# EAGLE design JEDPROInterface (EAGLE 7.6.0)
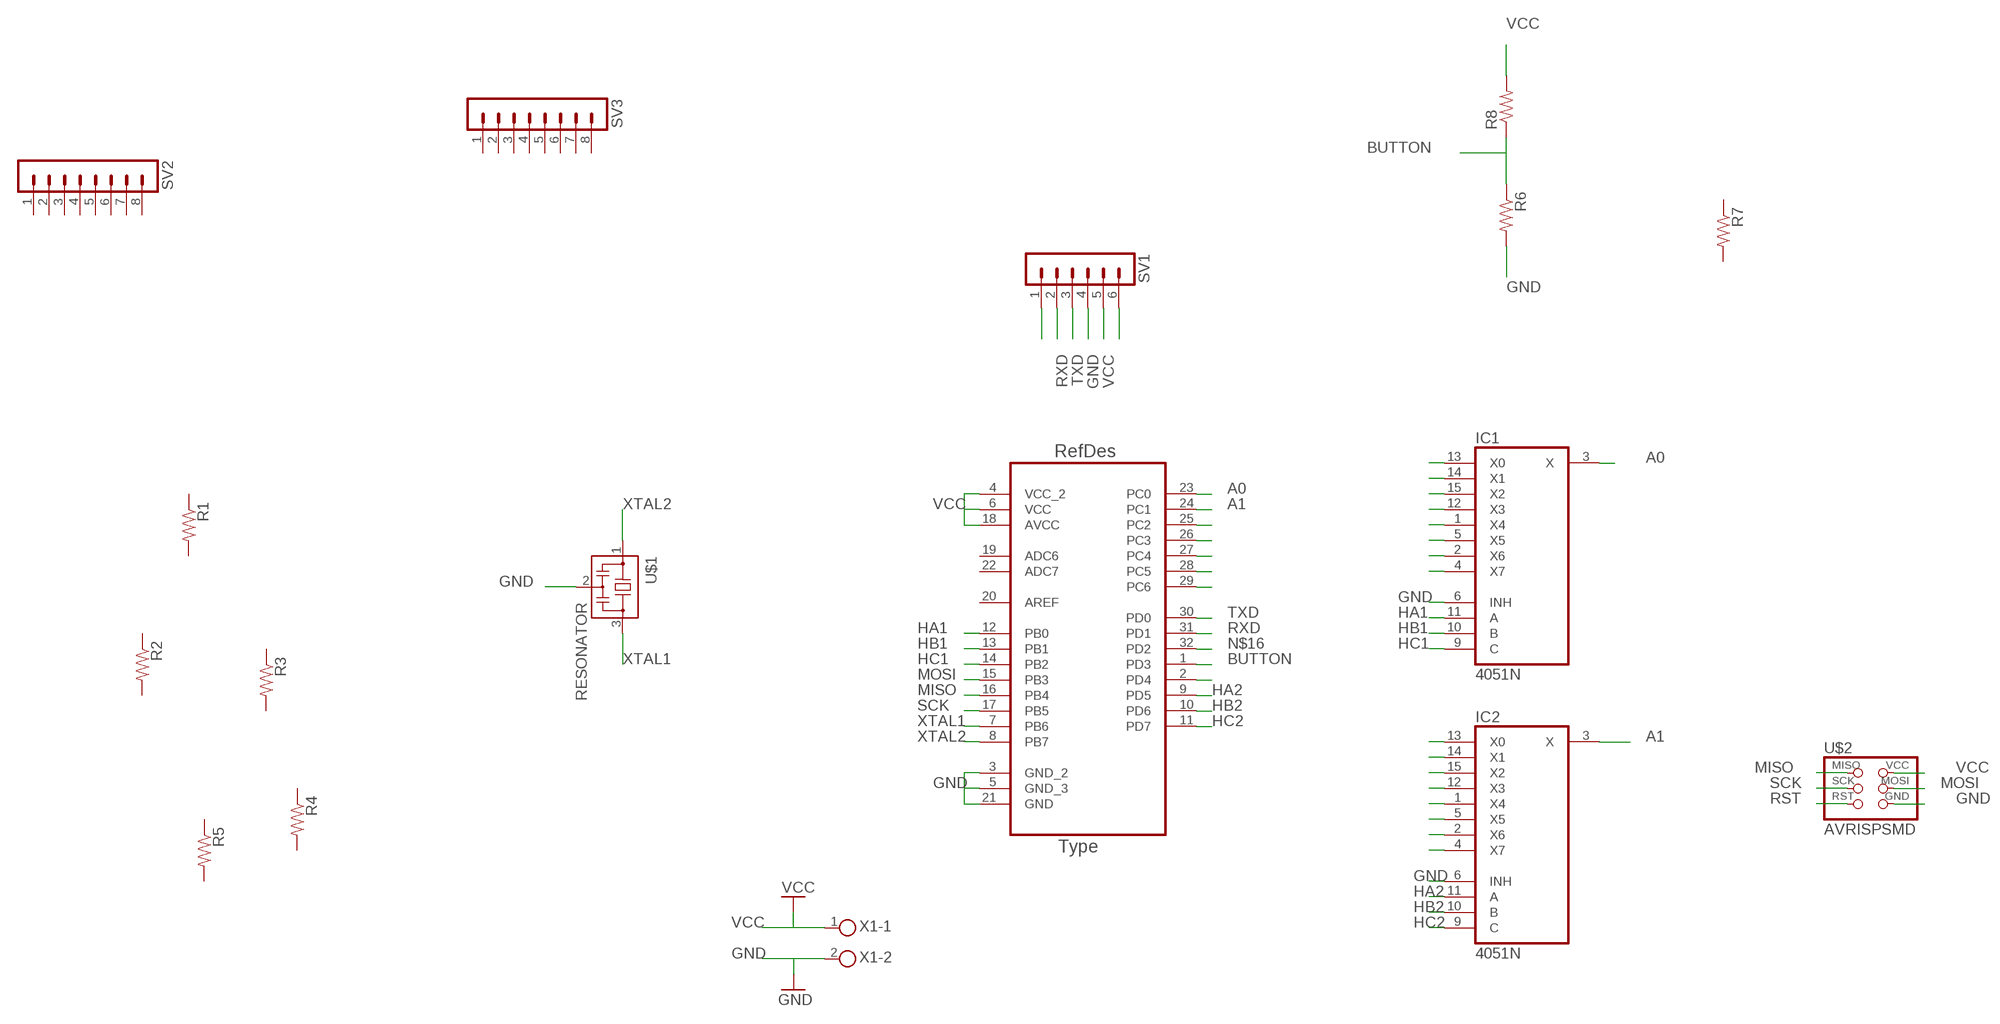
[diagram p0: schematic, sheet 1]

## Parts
IC1  4051N  [DIL16]
IC2  4051N  [DIL16]
R1  RES-US1206FAB  [R1206FAB]
R2  RES-US1206FAB  [R1206FAB]
R3  RES-US1206FAB  [R1206FAB]
R4  RES-US1206FAB  [R1206FAB]
R5  RES-US1206FAB  [R1206FAB]
R6  RES-US1206FAB  [R1206FAB]
R7  RES-US1206FAB  [R1206FAB]
R8  R-US_0204/7  [0204/7]
SV1  MA06-1  [MA06-1]
SV2  MA08-1  [MA08-1]
SV3  MA08-1  [MA08-1]
U1  ATMEGA328P-AU  [QFP80P900X900X120-32N]
U$1  RESONATOR  [EFOBM]
U$2  AVRISPSMD  [2X03SMD]
X1  AKL59-02  [2POL35]

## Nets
A0: IC1.3(X) U1.23(PC0)
A1: IC2.3(X) U1.24(PC1)
BUTTON: R6.1 R8.1 U1.1(PD3)
GND: IC1.6(INH) IC2.6(INH) R6.2 SV1.4 U1.3(GND_2) U1.5(GND_3) U1.21(GND) U$1.2 U$2.6(GND) X1.2
HA1: IC1.11(A) U1.12(PB0)
HA2: IC2.11(A) U1.9(PD5)
HB1: IC1.10(B) U1.13(PB1)
HB2: IC2.10(B) U1.10(PD6)
HC1: IC1.9(C) U1.14(PB2)
HC2: IC2.9(C) U1.11(PD7)
MISO: U1.16(PB4) U$2.1(MISO)
MOSI: U1.15(PB3) U$2.4(MOSI)
N$1: SV1.1
N$2: U1.28(PC5)
N$3: U1.27(PC4)
N$4: U1.26(PC3)
N$5: IC2.4(X7)
N$6: IC2.2(X6)
N$7: IC2.5(X5)
N$8: IC2.1(X4)
N$9: IC2.12(X3)
N$10: IC2.15(X2)
N$11: IC2.14(X1)
N$12: IC2.13(X0)
N$13: U1.25(PC2)
N$16: U1.32(PD2)
N$18: IC1.4(X7)
N$19: IC1.2(X6)
N$20: IC1.5(X5)
N$21: IC1.1(X4)
N$22: IC1.12(X3)
N$23: IC1.15(X2)
N$24: IC1.14(X1)
N$25: IC1.13(X0)
N$26: U1.2(PD4)
N$31: SV1.6
RST: U1.29(PC6) U$2.5(RST)
RXD: SV1.2 U1.31(PD1)
SCK: U1.17(PB5) U$2.3(SCK)
TXD: SV1.3 U1.30(PD0)
VCC: R8.2 SV1.5 U1.4(VCC_2) U1.6(VCC) U1.18(AVCC) U$2.2(VCC) X1.1
XTAL1: U1.7(PB6) U$1.3
XTAL2: U1.8(PB7) U$1.1
Unconnected: R1.1 R1.2 R2.1 R2.2 R3.1 R3.2 R4.1 R4.2 R5.1 R5.2 R7.1 R7.2 SV2.1 SV2.2 SV2.3 SV2.4 SV2.5 SV2.6 SV2.7 SV2.8 SV3.1 SV3.2 SV3.3 SV3.4 SV3.5 SV3.6 SV3.7 SV3.8 U1.19(ADC6) U1.20(AREF) U1.22(ADC7)

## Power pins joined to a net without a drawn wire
GND: IC1.8(GND) IC2.8(GND)
VCC: IC1.16(VCC) IC2.16(VCC)
VEE: IC1.7(VEE) IC2.7(VEE)

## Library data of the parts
IC1 IC2 = 40xx:4051: 8-channel ANALOG MULTIPLEXER
R1-R7 = fab:RES-US: Resistor (US Symbol)
R8 = rcl:R-US_: RESISTOR, American symbol
SV1 = con-lstb:MA06-1: PIN HEADER; OC_FARNELL: unknown; OC_NEWARK: unknown
SV2 SV3 = con-lstb:MA08-1: PIN HEADER; OC_FARNELL: unknown; OC_NEWARK: unknown
U1 = Atmel-ATMEGA328P-AU:ATMEGA328P-AU; DESCRIPTION: 8-bit Microcontroller with In-System Programmable Flash; MPN: ATMEGA328P-AU; OC_FARNELL: 1715486; OC_NEWARK: 14R4631; PACKAGE: TQFP-32; SUPPLIER: Atmel
U$1 = fab:RESONATOR
U$2 = fab:AVRISP
X1 = con-ria-59:AKL59-02: RIA Anschlussklemme Typ 59, Raster 3,5 mm, Polzahl 2

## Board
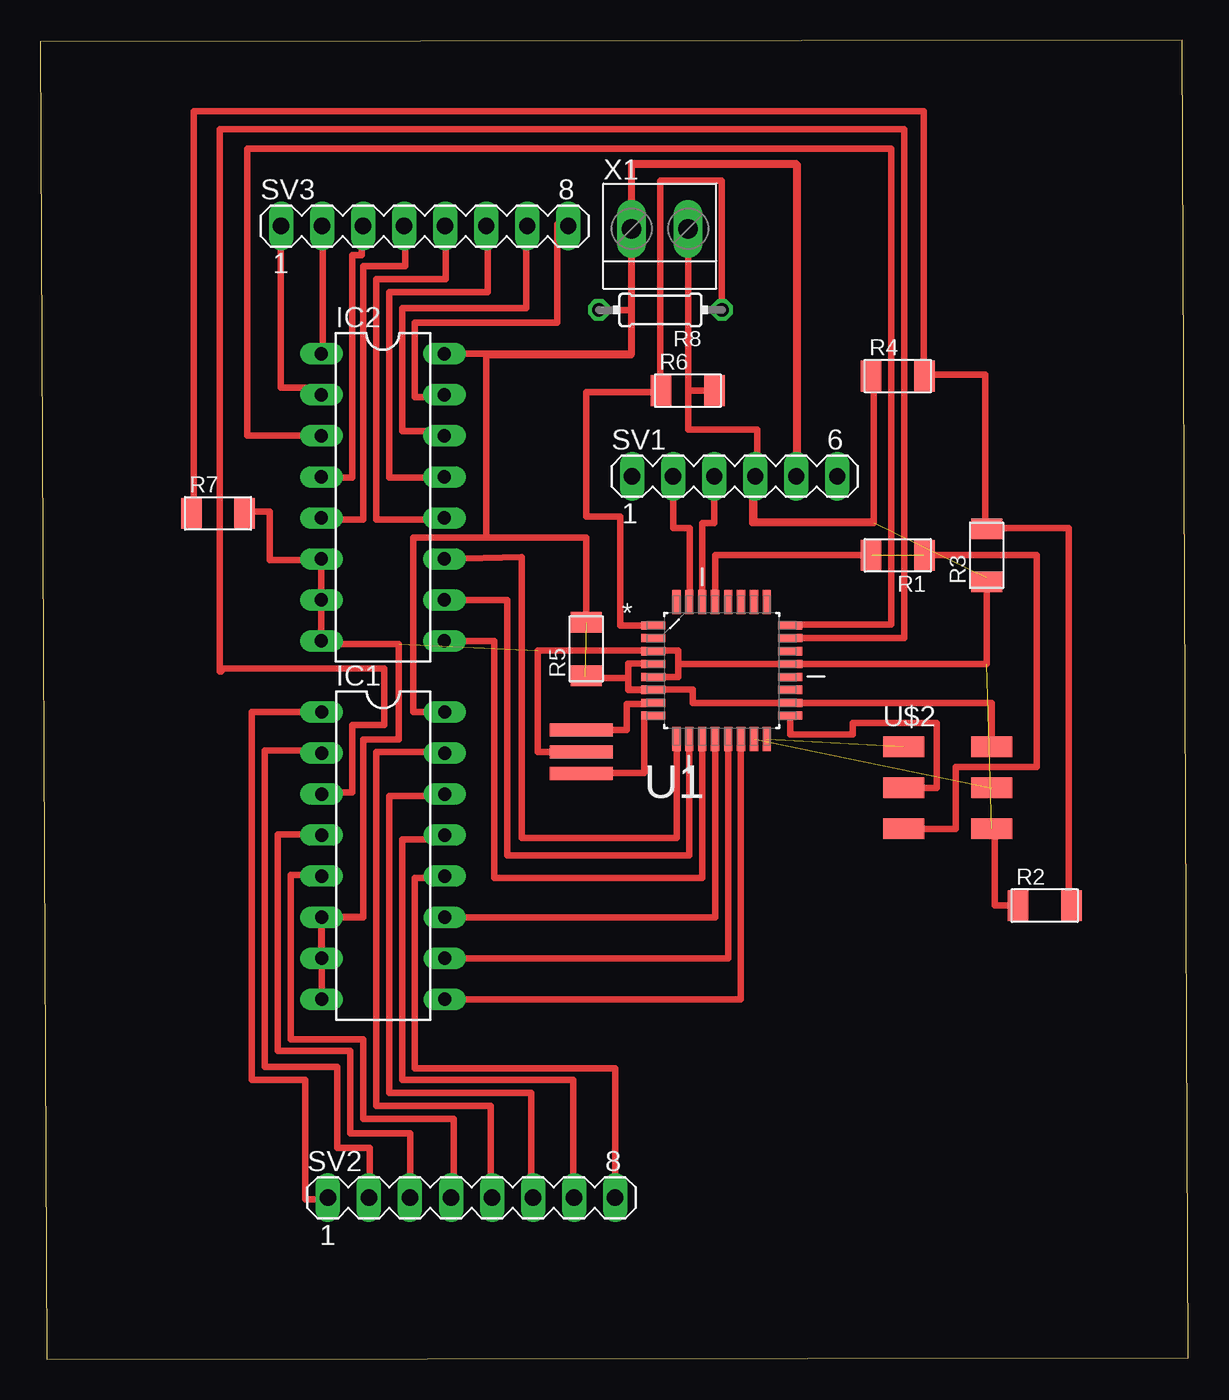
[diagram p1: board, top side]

Size 71.1 x 81.7 mm. Coordinates in mm from the lower left corner, seen from the top.
Outline: 0.4,0 71.1,0.1 70.7,81.7 0,81.6 0.4,0
Copper layers (1*16): Top 0.035mm / dielectric 1.5mm / Bottom 0.035mm
Design rules "default": minimum track width 10mil, minimum drill 24mil, track to track 8mil, track to pad 8mil, pad to pad 8mil, via to via 8mil, smd to smd 8mil, copper to edge 40mil, drill to drill 8mil, minimum pad ring 10mil, minimum via ring 8mil, stop-mask expansion 4mil, vias tented up to drill 0mil, thermal gap 10mil

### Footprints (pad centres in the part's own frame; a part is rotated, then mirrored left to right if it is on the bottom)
DIL16 = drill 0.813 long: 1 -8.89,-3.81; 2 -6.35,-3.81; 3 -3.81,-3.81; 4 -1.27,-3.81; 5 1.27,-3.81; 6 3.81,-3.81; 7 6.35,-3.81; 8 8.89,-3.81; 9 8.89,3.81; 10 6.35,3.81; 11 3.81,3.81; 12 1.27,3.81; 13 -1.27,3.81; 14 -3.81,3.81; 15 -6.35,3.81; 16 -8.89,3.81
R1206FAB = smd 1.27 x 1.905: 1 -1.651,0; 2 1.651,0
0204/7 = drill 0.813 octagon: 1 -3.81,0; 2 3.81,0
MA06-1 = drill 1.016 long: 1 -6.35,0; 2 -3.81,0; 3 -1.27,0; 4 1.27,0; 5 3.81,0; 6 6.35,0
MA08-1 = drill 1.016 long: 1 -8.89,0; 2 -6.35,0; 3 -3.81,0; 4 -1.27,0; 5 1.27,0; 6 3.81,0; 7 6.35,0; 8 8.89,0
QFP80P900X900X120-32N = smd 1.473 x 0.508: 1 -4.242,2.794; 2 -4.242,2.007; 3 -4.242,1.194; 4 -4.242,0.406; 5 -4.242,-0.406; 6 -4.242,-1.194; 7 -4.242,-2.007; 8 -4.242,-2.794; 17 4.242,-2.794; 18 4.242,-2.007; 19 4.242,-1.194; 20 4.242,-0.406; 21 4.242,0.406; 22 4.242,1.194; 23 4.242,2.007; 24 4.242,2.794 | smd 0.508 x 1.473: 9 -2.794,-4.242; 10 -2.007,-4.242; 11 -1.194,-4.242; 12 -0.406,-4.242; 13 0.406,-4.242; 14 1.194,-4.242; 15 2.007,-4.242; 16 2.794,-4.242; 25 2.794,4.242; 26 2.007,4.242; 27 1.194,4.242; 28 0.406,4.242; 29 -0.406,4.242; 30 -1.194,4.242; 31 -2.007,4.242; 32 -2.794,4.242
EFOBM = smd 0.8 x 3.9: 1 -1.35,0; 2 0,0; 3 1.35,0
2X03SMD = smd 2.54 x 1.27: 1 -2.54,2.54; 2 2.92,2.54; 3 -2.54,0; 4 2.92,0; 5 -2.54,-2.54; 6 2.92,-2.54
2POL35 = drill 1.2 long: 1 -1.75,0; 2 1.75,0

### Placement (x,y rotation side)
IC1  21.23,31.19 270 top
IC2  21.21,53.39 270 top
R1  53.1,49.8 180 top
R2  62.2,28.1 0 top
R3  58.6,49.8 90 top
R4  53.1,60.9 0 top
R5  33.8,44 90 top
R6  40.1,60 0 top
R7  11,52.4 0 top
R8  38.4,65 180 top
SV1  43,54.7 0 top
SV2  26.7,10 0 top
SV3  23.8,70.2 0 top
U1  42.19,42.66 0 top
U$1  33.5,37.62 90 top
U$2  56,35.4 0 top
X1  38.36,70.03 0 top

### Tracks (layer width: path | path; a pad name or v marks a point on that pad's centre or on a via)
A0
  Top 0.406: U1.23 53.5,44.67 53.5,76.2 11.1,76.2 11.1,42.6 11.2,42.6 11.2,42.8 21.3,42.8 21.3,39.3 19.3,39.3 19.3,35.1 17.42,35.1 IC1.3
A1
  Top 0.406: IC2.3 12.8,57.2 12.8,75 52.7,75 52.7,45.5 46.43,45.5 U1.24
BUTTON
  Top 0.406: U1.1 35.9,45.45 35.9,52.2 33.8,52.2 33.8,59.9 38.45,59.9 R6.1 38.4,60 38.4,73 42.21,73 R8.1
GND  (3 unrouted)
  Top 0.406: IC1.8 IC1.6 20,27.38 20,38.4 22.2,38.4 22.2,44.3 17.4,44.3 IC2.8 17.4,49.5 | 17.4,49.5 IC2.6 | U1.5 39.5,42.25 39.5,43.07 | 39.5,43.07 39.5,43.9 37.95,43.9 | 39.5,43.07 U1.21 58.6,43.07 58.6,48.4 | U$1.2 30.8,37.62 30.8,43.9 37.95,43.9 | 37.95,43.9 U1.3 | SV1.4 44.4,54.7 44.4,57.6 40.11,57.6 40.11,60 | 40.11,60 X1.2 | SV1.4 44.1,54.7 44.1,51.8 51.6,51.8 51.6,51.9 | 51.6,51.9 51.6,61 | SV1.4 44.2,54.7 44.2,51.9 51.6,51.9 | 17.4,49.5 14.2,49.5 14.2,52.5 12.5,52.5 12.5,52.6 | R6.2 40.11,60
HA1
  Top 0.406: IC1.11 41.78,27.38 U1.12
HA2
  Top 0.406: IC2.11 29.8,49.68 29.8,32.3 39.4,32.3 U1.9
HB1
  Top 0.406: IC1.10 42.6,24.84 U1.13
HB2
  Top 0.406: IC2.10 28.9,47.04 28.9,31.2 40.18,31.2 U1.10
HC1
  Top 0.406: IC1.9 43.38,22.3 U1.14
HC2
  Top 0.406: IC2.9 28.1,44.5 28.1,29.8 41,29.8 U1.11
MISO  (1 unrouted)
MOSI  (1 unrouted)
N$14
  Top 0.406: 17.5,30 15.5,30 15.5,19.8 20,19.8 20,14.9 25.6,14.9 25.6,9.9
N$15
  Top 0.406: 25.2,32.2 22.4,32.2 22.4,17.3 33,17.3 33,10
N$27
  Top 0.406: 24.9,34.9 21.6,34.9 21.6,16.5 30.4,16.5 30.4,13.8 30.4,13.7 30.4,10.1
N$28
  Top 0.406: 25,37.6 20.8,37.6 20.8,15.7 27.9,15.7 27.9,13.5
N$29
  Top 0.406: 59.1,32.5 59.1,28.1 60.6,28.1 60.6,28
N$30
  Top 0.406: 64.2,28.2 63.7,28.2 63.7,51.5 58.6,51.5 58.6,51.7
N$33
  Top 0.406: 25.2,59.6 23.2,59.6 23.2,64.2 32,64.2 32,70.1 32,70.2 32,70.3 32.7,70.3
N$34
  Top 0.406: 25.2,57.5 22.4,57.5 22.4,65.1 30.1,65.1 30.1,70.2
N$35
  Top 0.406: 25.1,54.6 21.6,54.6 21.6,66.1 27.7,66.1 27.7,70.2
N$36
  Top 0.406: 25,52 20.8,52 20.8,66.9 25.1,66.9 25.1,70.2
N$37
  Top 0.406: 17.3,52 20,52 20,67.7 22.6,67.7 22.6,70
N$38
  Top 0.406: 17.4,54.6 19.3,54.6 19.3,68.4 19.9,68.4 19.9,70.2
N$39
  Top 0.406: 17.5,62.3 17.5,70.4
N$40
  Top 0.406: 17.5,60.2 14.9,60.2 14.9,70.5
N$41
  Top 0.406: 25,29.8 23.2,29.8 23.2,18 35.6,18 35.6,13.7 35.6,13.6 35.6,9.9
N$42
  Top 0.406: 27.9,13.4 27.9,9.9
N$43
  Top 0.406: 17.6,32.5 14.7,32.5 14.7,19.1 19.2,19.1 19.2,14 22.9,14 22.9,10
N$44
  Top 0.406: 17.6,37.7 13.9,37.7 13.9,18.1 18.4,18.1 18.4,13.1 20.4,13.1 20.4,10.1
N$45
  Top 0.406: 17.4,40.1 13.1,40.1 13.1,17.3 16.4,17.3 16.4,9.9 17.7,9.9 17.7,10.1
N$46
  Top 0.406: 9.5,53 9.5,77.3 54.7,77.3 54.7,61 58.5,61 58.5,51.4 58.7,51.4
RST  (1 unrouted)
  Top 0.406: U$2.5 56.7,32.86 56.7,36.7 61.7,36.7 61.7,49.8 54.7,49.8 | U1.29 41.78,49.8 51.5,49.8
RXD
  Top 0.406: U1.31 40.2,46.9 40.2,51.5 39.19,51.5 SV1.2
SCK
  Top 0.406: U$2.3 55.5,35.4 55.5,39.4 50.3,39.4 50.3,38.7 46.43,38.7 U1.17
TXD
  Top 0.406: U1.30 41,51.8 41.73,51.8 SV1.3
VCC  (1 unrouted)
  Top 0.406: U$2.2 58.92,40.65 U1.18 40.4,40.65 40.4,41.5 37.95,41.5 | 37.95,41.5 U1.6 36.4,41.47 36.4,41.5 | 36.4,42.2 36.4,43.1 37.95,43.1 U1.4 | 25.02,62.3 IC2.16 27.6,62.28 | 27.6,62.28 36.61,62.28 X1.1 36.61,74 46.9,74 46.9,54.7 SV1.5 | 27.6,62.2 27.6,62.28 | 27.6,50.9 23.1,50.9 23.1,40.08 IC1.16 | 27.6,50.9 27.6,62.2 | 27.6,62.2 36.6,62.2 36.6,64.6 36.6,65 | 36.6,65 36.6,74.1 46.8,74.1 46.8,54.8 | 37.95,41.5 36.4,41.5 | 36.4,41.5 36.4,42.2 | 36.4,42.2 33.7,42.2 33.7,42.3 | 27.6,50.9 33.8,50.9 33.8,45.6 | R8.2 36.6,65
VEE
  Top 0.406: IC1.7 17.4,24.84 17.4,27.4 20,27.4 20,38.4 22.2,38.4 22.2,44.3 17.4,44.3 IC2.7
XTAL1
  Top 0.406: U$1.3 36.3,38.97 36.3,40.6 37.95,40.6 U1.7
XTAL2
  Top 0.406: U1.8 37.4,39.87 37.4,36.3 32.4,36.3 U$1.1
